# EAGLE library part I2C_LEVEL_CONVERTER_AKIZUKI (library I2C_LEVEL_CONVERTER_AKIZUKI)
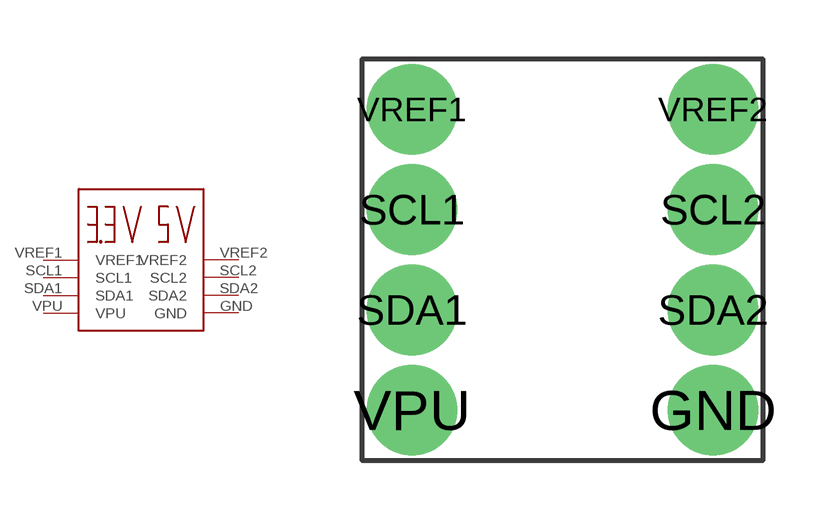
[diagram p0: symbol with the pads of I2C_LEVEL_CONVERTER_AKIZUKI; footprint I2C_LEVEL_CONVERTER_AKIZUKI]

Designator prefix I2C_LEVEL

## I2C_LEVEL_CONVERTER_AKIZUKI  [I2C_LEVEL_CONVERTER_AKIZUKI]
GND  GND
SCL1  SCL1
SCL2  SCL2
SDA1  SDA1
SDA2  SDA2
VPU  VPU
VREF1  VREF1
VREF2  VREF2

## Footprint I2C_LEVEL_CONVERTER_AKIZUKI (pad centres in mm)
drill 1 pad 2.3: GND 7.62,0; SCL1 0,5.08; SCL2 7.62,5.08; SDA1 0,2.54; SDA2 7.62,2.54; VPU 0,0; VREF1 0,7.62; VREF2 7.62,7.62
